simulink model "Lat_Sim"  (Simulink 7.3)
settings: Solver=ode45  StartTime=0.0  StopTime=20  RelTol=1e-3
undefined symbols (not defined in the file or in its folder): Ali, Bli, Cli, Dli, Kpr

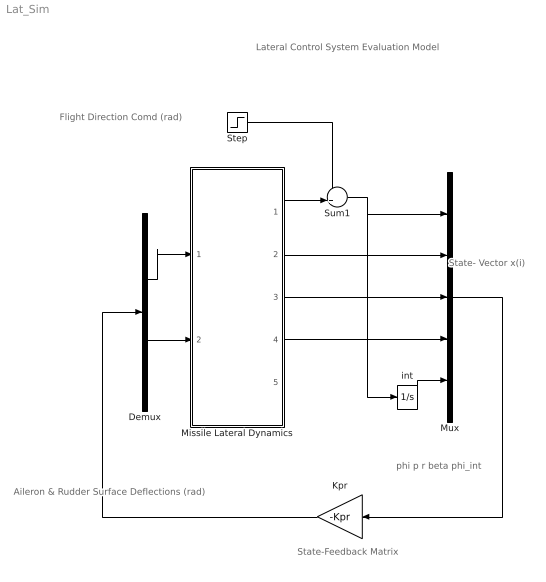
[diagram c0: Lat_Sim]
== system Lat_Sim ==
  note: phi p r beta phi_int
  note: Flight Direction Comd (rad)
  note: State- Vector x(i)
  note: Aileron & Rudder Surface Deflections (rad)
  note: State-Feedback Matrix
  note: Lateral Control System Evaluation Model
  Demux : Demux  Outputs=2
  Kpr : Gain  Gain=-Kpr  Multiplication=Matrix(K*u)  ParameterDataType=fixdt(1, 16)  ParameterScaling=2^0  OutDataType=fixdt(1, 16)  OutScaling=2^0
  Missile Lateral Dynamics : Subsystem
  Mux : Mux  Inputs=5
  Step : Step  Time=0  SampleTime=0
  Sum1 : Sum  Inputs=-+|  OutDataType=fixdt(1, 16)  OutScaling=2^0
  int : Integrator
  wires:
  Demux/2 -> Missile Lateral Dynamics/2(DR_mix)
  Kpr/1 -> Demux/1
  Mux/1 -> Kpr/1
  Step/1 -> Sum1/1
  Demux/1 -> Missile Lateral Dynamics/1(DP_mix)
  Missile Lateral Dynamics/2(p) -> Mux/2
  Missile Lateral Dynamics/3(r) -> Mux/3
  Missile Lateral Dynamics/4(beta) -> Mux/4
  Missile Lateral Dynamics/1(phi) -> Sum1/2
  Sum1/1 -> Mux/1, int/1
  int/1 -> Mux/5

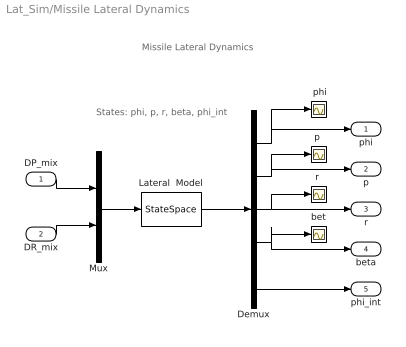
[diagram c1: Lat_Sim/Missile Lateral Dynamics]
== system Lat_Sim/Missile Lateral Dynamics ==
  note: Missile Lateral Dynamics
  note: States: phi, p, r, beta, phi_int
  DP_mix : Inport  OutDataType=sfix(16)  OutScaling=2^0
  DR_mix : Inport  Port=2  OutDataType=sfix(16)  OutScaling=2^0
  " phi" : Scope
  Demux : Demux  Outputs=5
  Lateral  Model : StateSpace  A=Ali  B=Bli  C=Cli  D=Dli
  Mux : Mux  Inputs=2
  bet : Scope
  "p " : Scope
  "r " : Scope
  phi : Outport  OutDataType=sfix(16)  OutScaling=2^0
  p : Outport  Port=2  OutDataType=sfix(16)  OutScaling=2^0
  r : Outport  Port=3  OutDataType=sfix(16)  OutScaling=2^0
  beta : Outport  Port=4  OutDataType=sfix(16)  OutScaling=2^0
  phi_int : Outport  Port=5  OutDataType=sfix(16)  OutScaling=2^0
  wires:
  Mux/1 -> Lateral  Model/1
  Lateral  Model/1 -> Demux/1
  DP_mix/1 -> Mux/1
  DR_mix/1 -> Mux/2
  Demux/1 -> phi/1, " phi"/1
  Demux/2 -> p/1, "p "/1
  Demux/3 -> r/1, "r "/1
  Demux/4 -> beta/1, bet/1
  Demux/5 -> phi_int/1
